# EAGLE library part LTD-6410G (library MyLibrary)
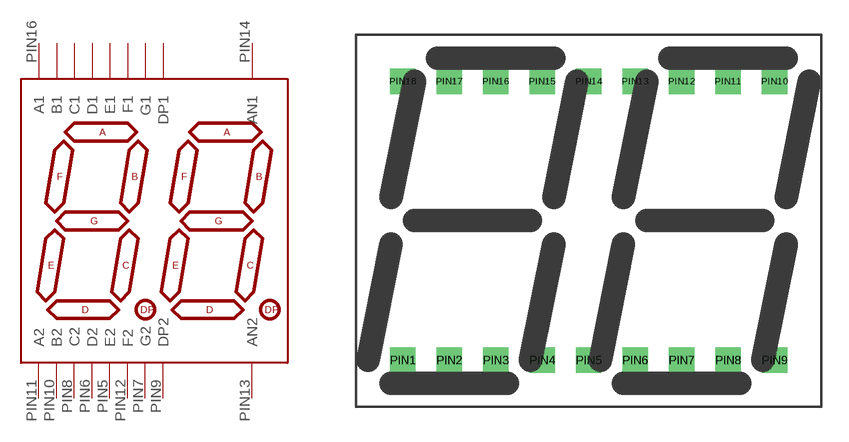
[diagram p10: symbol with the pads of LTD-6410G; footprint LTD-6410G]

Designator prefix -

## LTD-6410G  [LTD-6410G]
PIN1  E1
PIN2  D1
PIN3  C1
PIN4  DP1
PIN5  E2
PIN6  D2
PIN7  G2
PIN8  C2
PIN9  DP2
PIN10  B2
PIN11  A2
PIN12  F2
PIN13  AN2
PIN14  AN1
PIN15  B1
PIN16  A1
PIN17  G1
PIN18  F1

## Footprint LTD-6410G (pad centres in mm)
drill 0.9 square: PIN1 -10.16,-7.62; PIN2 -7.62,-7.62; PIN3 -5.08,-7.62; PIN4 -2.54,-7.62; PIN5 0,-7.62; PIN6 2.54,-7.62; PIN7 5.08,-7.62; PIN8 7.62,-7.62; PIN9 10.16,-7.62; PIN10 10.16,7.62; PIN11 7.62,7.62; PIN12 5.08,7.62; PIN13 2.54,7.62; PIN14 0,7.62; PIN15 -2.54,7.62; PIN16 -5.08,7.62; PIN17 -7.62,7.62; PIN18 -10.16,7.62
